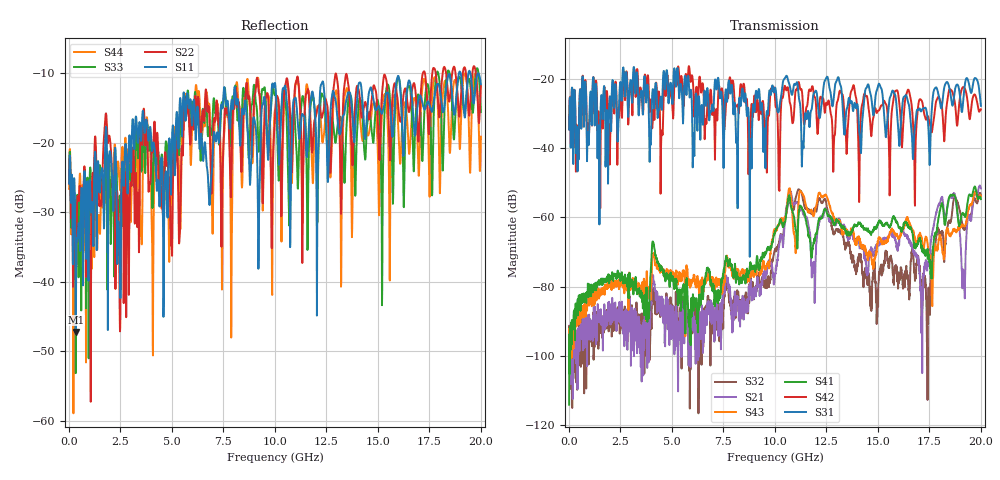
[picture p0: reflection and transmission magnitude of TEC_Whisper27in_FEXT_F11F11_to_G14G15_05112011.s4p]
! Tyco Electronics
! F11F12-G14G15_FEXT
!! PART DESCRIPTION: Whisper 27in Megtron 6 VLP-HVLP-VLP Channel Model, bulkhead 2.4mm test pts
!! MODEL DESCRIPTION: System 4-port S-parameter
!! MODEL STATUS: Measured
!! MODEL GEOMETRY: Channel Model
!! MODEL FREQUENCY RANGE: DC to 20.000 GHz in 10.000 MHz frequency steps
!! MODEL EDGE RATE LIMITATION: 25.50 ps (Using conservative 0.5/Fmax rule of thumb)
!! TIME-DOMAIN TRANSFORM CAUTIONS:
!! 1.) Do not simulate transient edge rates faster than the number listed above.  Edge rates faster than this number
!!  contain significant spectral content at frequencies above the model's highest frequency.
!! 2.) Even when simulating edge rates that are slower than the number listed above, be aware that the best time
!!  resolution possible with a direct iFFT is (1 / 2Fmax).  As a result, time resolution is typically not adequate
!!  for most time-domain simulations unless tricks such as windowing are used to minimize leakage and aliasing.
!! 3.) Because the model has a uniform frequency step, a direct iFFT will result in an impulse that that has a time
!!  length given by either (1 / Fstep) or (1 / 2Fstep), depending on the transform being used.  Care has been taken
!!  in selecting the frequency step to ensure a settled impulse response for the model.  Therefore, convolution with
!!  the model's impulse response should present no issues.  However, if directly concatenating s-parameter models
!!  in the frequency domain a user must either interpolate necessary interim frequencies or complete impulse response
!!  zero-padding.  Impulse response zero-padding is more difficult, but more accurate.
!! PORT DEFINITIONS:
!! Port  1  ----->  Side A  F11  G14  Side B  <-----  Port  2
!! Port  3  ----->  Side A  F12  G15  Side B  <-----  Port  4
! Point-to-Point link (differential)  !
! Connectors:  !
!  1: STRADA Whisper  !
! Materials:  !
!  Backplane: Megtron-6 HVLP  !
!  Daughtercard: Megtron-6 VLP  !
! Stack-up:  !
!  Backplane: 20 layers, 200mil thick  !
!  Daughtercard: 14 layers, 110mil thick  !
! Trace Length:  !
!  Backplane: 17in  !
!  Daightercards: 5in  !
! Trace Width:  !
!  Backplane: 8-13-8 mils  !
!  Daughtercards: 6-9-6 mils  !
! Geometry:  !
!  Backplane: Stripline  !
!  Daughtercards: Stripline  !
! Freq. Range: 0 GHz - 20 GHz  !
! Note1: non-mixed-mode s-parameters  !
! Note2: channel includes 2.4mm test points  !
! Created Wed May 11 14:41:25 2011
! 4 Port Network Data from SP1.SP block
! freq  magS11  angS11  magS12  angS12  magS13  angS13  magS14  angS14
!  magS21  angS21  magS22  angS22  magS23  angS23  magS24  angS24
!  magS31  angS31  magS32  angS32  magS33  angS33  magS34  angS34
!  magS41  angS41  magS42  angS42  magS43  angS43  magS44  angS44
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# hz S ma R 50
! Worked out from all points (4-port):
!   2000 points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, 10 MHz to 20 GHz, reference 50 ohm
!   strongest paths, dB at 10 MHz, 5.01 GHz, 10.01 GHz, 15.01 GHz, 20 GHz:
!     S31: -34.6, -25.9, -22.5, -21.9, -27.7
!     S42: -34.5, -26.8, -26.0, -29.1, -28.8
!     S41: -114.1, -77.8, -64.4, -61.8, -54.7
!     S43: -99.1, -76.3, -63.4, -67.2, -53.9
!     S21: -98.4, -94.3, -76.4, -67.7, -51.6
!     S32: -94.6, -85.1, -69.4, -85.8, -53.6
!   lowest |S11| = -47.2 dB at 330 MHz (marker M1), VSWR 1.01, Z = 49.6 + j0.0067 ohm
!   |S11| at or under -10 dB: start of sweep to 18.94 GHz; 19.02 GHz to 19.4 GHz (382.1 MHz wide, 1.99 % of centre); 19.49 GHz to end of sweep
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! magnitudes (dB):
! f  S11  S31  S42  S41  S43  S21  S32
! 10 MHz  -25.9  -34.6  -34.5  -114.1  -99.1  -98.4  -94.6
! 330 MHz  -47.2  -38.4  -41.4  -84.9  -88.0  -96.1  -106.6
! 9.29 GHz  -22.0  -27.9  -26.5  -72.6  -75.6  -80.8  -78.6
! 10.77 GHz  -27.8  -23.4  -27.8  -56.7  -53.3  -52.7  -54.9
! 18.68 GHz  -15.7  -25.8  -25.1  -53.5  -63.4  -53.3  -55.0
! 19.15 GHz  -13.9  -25.5  -22.3  -59.1  -62.4  -75.2  -63.3
! 20 GHz  -11.6  -27.7  -28.8  -54.7  -53.9  -51.6  -53.6
